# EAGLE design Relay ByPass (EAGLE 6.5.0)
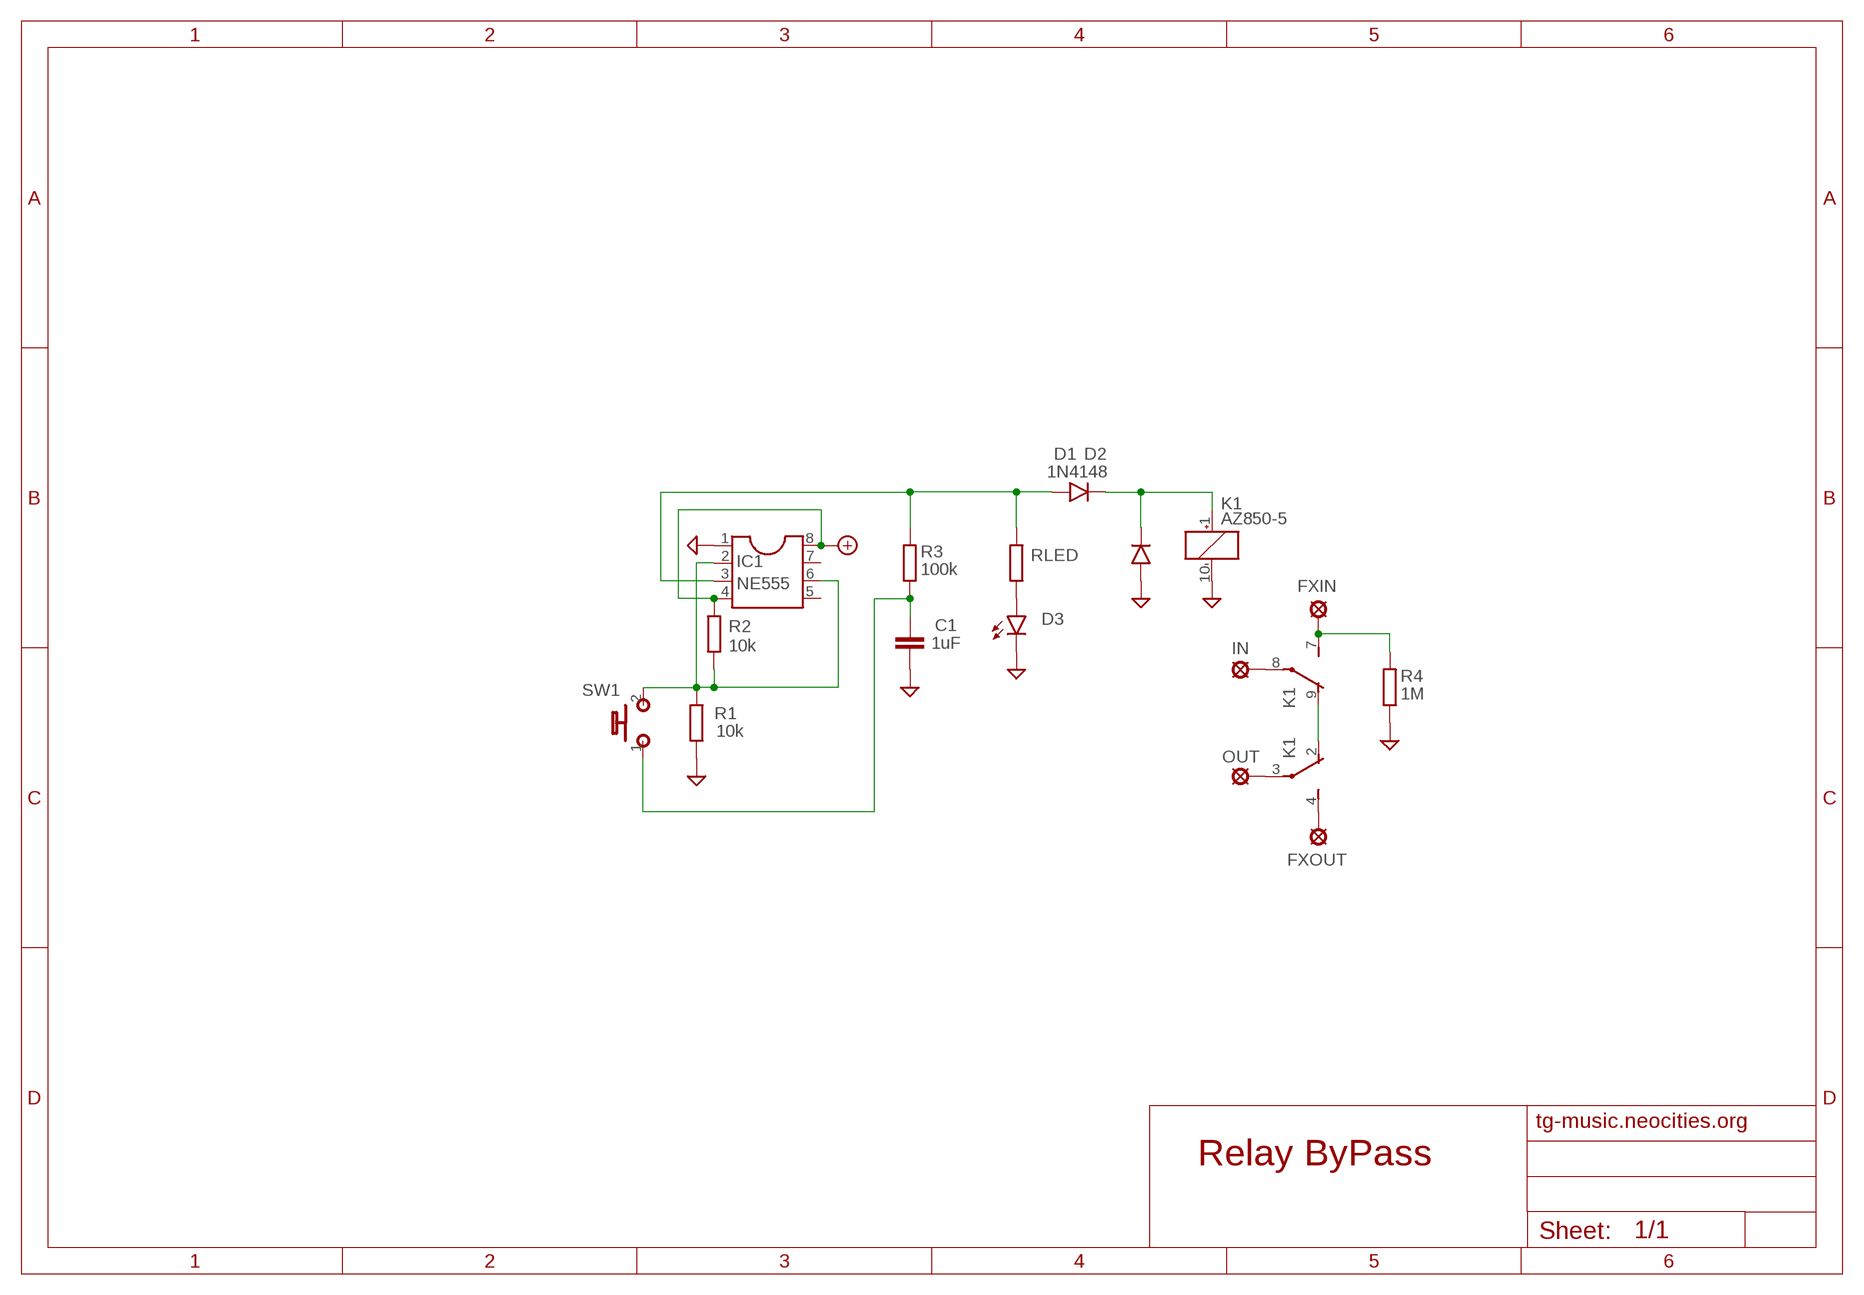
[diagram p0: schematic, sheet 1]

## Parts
+9V  +9V(T)1  [ROUND]
C1  1uF  C-EUC0805  [C0805]
D1  1N4148  1N400X.1  [DO41-1]
D2  1N4005  1N400X.1  [DO41-1]
D3  LED3MM  [LED3MM]
FXIN  LSP10  [LSP10]
FXOUT  LSP10  [LSP10]
GND  GND  GND(T)1  [ROUND]
IC1  NE555  DIL8D  [SO08]
IN  LSP10  [LSP10]
K1  AZ850-5  TQ2-5V  [TQ2]
OUT  LSP10  [LSP10]
R1  10k  R-EU_R0805  [R0805]
R2  10k  R-EU_R0805  [R0805]
R3  100k  R-EU_R0805  [R0805]
R4  1M  R-EU_R0805  [R0805]
RLED  R-EU_R0805  [R0805]
SW1  BYPASS  MOMENTARY  [SPST]

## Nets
+9V: +9V.1(+9V) IC1.4 IC1.8 R2.2
GND: C1.2 D2.A D3.K(C) GND.1(GND) IC1.1 K1.10(_:-) R1.1 R4.1
N$1: K1.2(1:O) K1.9(2:O)
N$2: FXIN.MP K1.7(2:S) R4.2
N$3: IN.MP K1.8(2:P)
N$4: K1.3(1:P) OUT.MP
N$5: FXOUT.MP K1.4(1:S)
N$6: D3.A RLED.1
N$22: IC1.2 IC1.6 R1.2 R2.1 SW1.2(S)
N$24: D1.A IC1.3 R3.2 RLED.2
N$25: C1.1 R3.1 SW1.1(P)
N$26: D1.C D2.C K1.1(_:+)
Unconnected: IC1.5 IC1.7

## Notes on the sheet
- tg-music.neocities.org

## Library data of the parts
+9V = Virransyöttö:+9V(T): +9V Voltage Supply
C1 = rcl:C-EU: CAPACITOR, European symbol
D1 D2 = Diodit:1N400X: Rectifier Diodes
D3 = Diodit:LED
FXIN FXOUT IN OUT = Padit:LSP10: SOLDER PAD
GND = Virransyöttö:GND(T): Ground
IC1 = ic-package:DIL8: Dual In Line / Socket
K1 = relay:TQ2?*: LOW PROFILE 2 FORM C RELAY NAiS Source: http://www.mew-europe.com/.. en_ds_61020_0001.pdf Source: http://www.mew-europe.com/.. en_ds_61020_0004.pdf; MF: AROMAT/ MATSUSHITA; MPN: TQ2-5V; OC_FARNELL: 1175716; OC_NEWARK: 64K3200
R1-R4 RLED = rcl:R-EU_: RESISTOR, European symbol
SW1 = Kytkimet:MOMENTARY

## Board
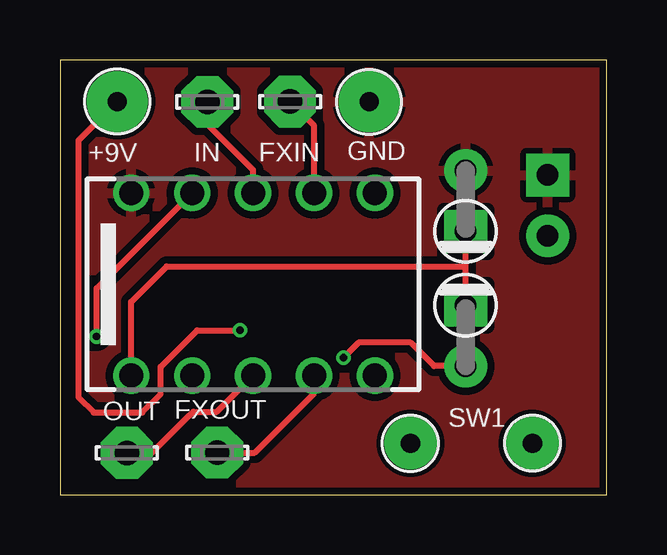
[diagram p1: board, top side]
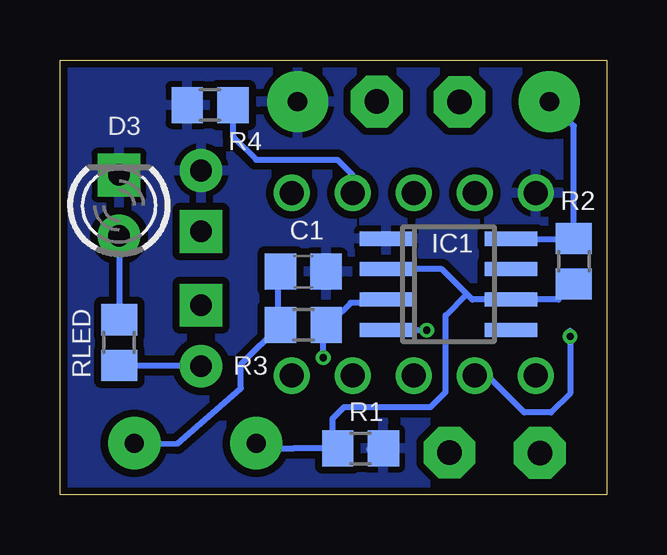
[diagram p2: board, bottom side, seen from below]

Size 22.78 x 18.14 mm. Coordinates in mm from the lower left corner, seen from the top.
Outline: 0,0 22.78,0 22.78,18.14 0,18.14 0,0
Copper layers (1*16): Top 0.035mm / dielectric 1.5mm / Bottom 0.035mm
Design rules "ITEADstudio": minimum track width 10mil, minimum drill 12mil, track to track 12mil, track to pad 12mil, pad to pad 12mil, via to via 12mil, smd to smd 0mil, copper to edge 12mil, drill to drill 12mil, minimum pad ring 10mil, minimum via ring 6mil, stop-mask expansion 4mil, vias tented up to drill 100mil, thermal gap 10mil

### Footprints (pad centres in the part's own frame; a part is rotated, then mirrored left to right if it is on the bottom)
ROUND = drill 0.8 pad 2.54: 1 0,0
C0805 = smd 1.3 x 1.5: 1 -0.95,0; 2 0.95,0
DO41-1 = drill 0.9 pad 1.778: A 1.27,0 | drill 0.9 pad 1.778 square: C -1.27,0
LED3MM = drill 0.9 pad 1.778: A -1.27,0 | drill 0.9 pad 1.778 square: K 1.27,0
LSP10 = drill 1.016 pad 2.159 octagon: MP 0,0
SO08 = smd 0.6 x 2.2: 1 -1.905,-2.6; 2 -0.635,-2.6; 3 0.635,-2.6; 4 1.905,-2.6; 5 1.905,2.6; 6 0.635,2.6; 7 -0.635,2.6; 8 -1.905,2.6
TQ2 = drill 1: 1 -5.08,-3.81; 2 -2.54,-3.81; 3 0,-3.81; 4 2.54,-3.81; 5 5.08,-3.81; 6 5.08,3.81; 7 2.54,3.81; 8 0,3.81; 9 -2.54,3.81; 10 -5.08,3.81
R0805 = smd 1.3 x 1.5: 1 -0.95,0; 2 0.95,0
SPST = drill 0.8 pad 2.184: 1 -2.54,0; 2 2.54,0

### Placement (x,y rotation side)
+9V  2.39,16.4 0 top
C1  12.64,9.3 0 bottom
D1  16.9,6.64 270 top
D2  16.9,12.25 90 top
D3  20.32,12.07 90 bottom
FXIN  9.58,16.4 0 top
FXOUT  6.55,1.76 0 top
GND  12.88,16.39 0 top
IC1  6.59,8.78 270 bottom
IN  6.14,16.39 0 top
K1  8.04,8.78 0 top
OUT  2.79,1.74 0 top
R1  10.26,1.93 180 bottom
R2  1.37,9.74 90 bottom
R3  12.64,7.08 0 bottom
R4  16.53,16.25 0 bottom
RLED  20.32,6.35 270 bottom
SW1  17.15,2.15 180 top

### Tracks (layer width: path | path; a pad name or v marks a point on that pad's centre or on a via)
+9V  (via drill 0.3)
  Top 0.254: v7.5,6.86 5.72,6.86 4.19,5.33 4.19,4.19 3.43,3.43 1.4,3.43 0.76,4.06 0.76,14.77 +9V.1
  Bottom 0.254: IC1.8 3.81,10.67 1.52,10.67 R2.2 1.37,15.38 +9V.1 | v7.5,6.86 9.14,6.86 IC1.4
GND
  Bottom 0.254: R1.1 9.91,1.91 9.87,1.83
  pour Bottom: 0,0 0,18.13 22.74,18.13 22.74,0
  pour Top: 0,0 0,18.13 22.76,18.13 22.76,0
N$1  (via drill 0.3)
  Top 0.254: v1.52,6.6 1.52,8.61 K1.9
  Bottom 0.254: v1.52,6.6 1.52,6.84 1.52,4.23 2.32,3.43 3.43,3.43 4.95,4.95 5.33,4.95 K1.2
N$2
  Top 0.254: K1.7 10.59,15.4 FXIN.MP
  Bottom 0.254: R4.2 15.58,14.94 14.61,13.97 11.22,13.97 10.59,13.34 K1.7
N$3
  Top 0.254: K1.8 8.05,13.55 6.14,15.45 IN.MP
N$4
  Top 0.254: OUT.MP 3.82,1.74 5.24,3.16 | 5.24,3.16 | 5.24,3.16 5.38,3.3 5.4,3.3 5.56,3.47 6.54,3.47 K1.3
N$5
  Top 0.254: K1.4 10.59,4.24 8.11,1.76 FXOUT.MP
N$6
  Bottom 0.254: D3.A RLED.1
N$22
  Bottom 0.254: 5.83,8.37 5.6,8.14 IC1.6 2.01,8.14 R2.1 | 5.83,8.37 6.87,9.41 IC1.2 | 5.83,8.37 6.71,7.48 6.71,4.29 7.34,3.65 10.95,3.65 11.43,3.18 11.43,2.15 R1.2 13.06,1.93 14.3,1.94 SW1.2
N$24  (via drill 0.3)
  Top 0.254: D1.A 15.59,5.37 14.61,6.35 12.45,6.35 v11.81,5.72
  Bottom 0.254: IC1.3 9.53,8 10.67,8 11.43,7.24 R3.2 11.81,6.86 v11.81,5.72 | RLED.2 16.9,5.4 D1.A
N$25
  Bottom 0.254: C1.1 13.72,9.14 13.72,7.24 R3.1 15.24,5.44 15.24,4.45 17.9,2.13 SW1.1
N$26
  Top 0.254: K1.1 2.97,8.05 4.45,9.53 16.9,9.53 | D1.C 16.9,9.53 | 16.9,9.53 D2.C | D2.C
